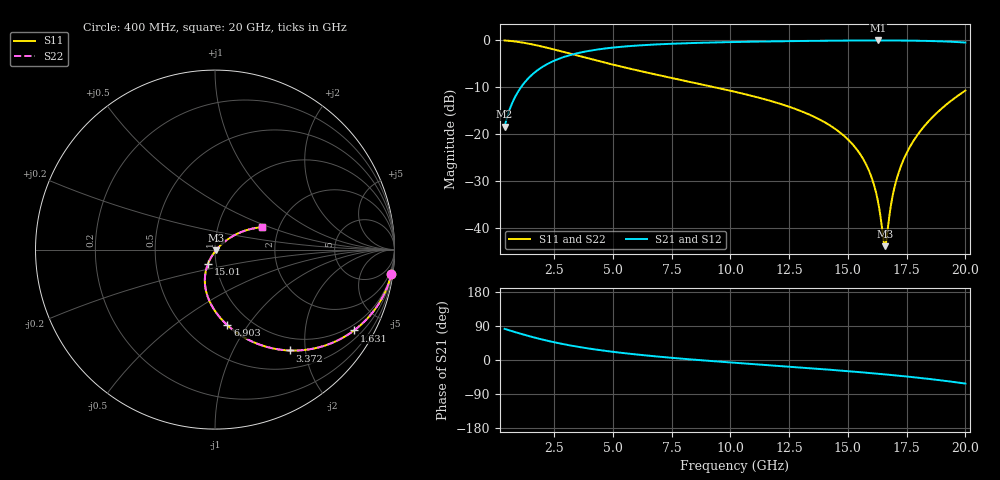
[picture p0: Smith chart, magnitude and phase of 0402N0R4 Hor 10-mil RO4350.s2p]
# GHz S MA R 50
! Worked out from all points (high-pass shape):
!   1960 points, 400 MHz to 20 GHz, reference 50 ohm
!   highest |S21| = -0.06 dB at 16.29 GHz (marker M1); lowest = -18.4 dB at 400 MHz (marker M2)
!   |S21| within 3 dB of the highest: 3.269 GHz to end of sweep
!   lowest |S11| = -43.8 dB at 16.58 GHz (marker M3), VSWR 1.01, Z = 50.5 - j0.407 ohm
!   |S11| at or under -10 dB: 9.329 GHz to end of sweep
!   |S22| runs from -43.8 to -0.1 dB; largest |S21 - S12| = 0
!   S11 on the Smith chart (normalised r, x): 400 MHz: 1, -15; 1.631 GHz: 0.78, -3.55; 3.372 GHz: 0.78, -1.71; 6.903 GHz: 0.78, -0.81; 15.01 GHz: 0.91, -0.15; 20 GHz: 1.64, +0.45
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0.4  0.9927 -7.9  0.1205 82.1  0.1205 82.1  0.9927 -7.9
0.9202654  0.9631 -17.8  0.2689 72.2  0.2689 72.2  0.9631 -17.8
1.630628  0.8962 -30.2  0.4432 59.8  0.4432 59.8  0.8962 -30.2
3.371516  0.6993 -53.5  0.7138 36.4  0.7138 36.4  0.6993 -53.5
3.671669  0.6683 -56.6  0.7428 33.3  0.7428 33.3  0.6683 -56.6
5.132414  0.5401 -69.2  0.8401 20.6  0.8401 20.6  0.5401 -69.2
6.903318  0.4272 -80.7  0.9022 9.1  0.9022 9.1  0.4272 -80.7
6.943338  0.425 -80.9  0.9032 8.9  0.9032 8.9  0.425 -80.9
10.205  0.2823 -96.9  0.9563 -7.4  0.9563 -7.4  0.2823 -96.9
13.46667  0.1573 -110.6  0.983 -22.1  0.983 -22.1  0.1573 -110.6
15.00745  0.08774 -116.2  0.9905 -29.5  0.9905 -29.5  0.08774 -116.2
15.80786  0.04596 -116.6  0.9926 -33.7  0.9926 -33.7  0.04596 -116.6
16.078  0.03085 -114.1  0.993 -35.1  0.993 -35.1  0.03085 -114.1
16.28811  0.01891 -107.4  0.993 -36.3  0.993 -36.3  0.01891 -107.4
16.50822  0.007775 -72.6  0.9929 -37.5  0.9929 -37.5  0.007775 -72.6
16.57825  0.00644 -38.8  0.9929 -38.0  0.9929 -38.0  0.00644 -38.8
16.73834  0.01207 17.9  0.9926 -38.9  0.9926 -38.9  0.01207 17.9
16.89842  0.02165 31.9  0.9923 -39.8  0.9923 -39.8  0.02165 31.9
17.09852  0.03476 37.3  0.9917 -41.0  0.9917 -41.0  0.03476 37.3
17.69883  0.07773 39.4  0.9884 -44.8  0.9884 -44.8  0.07773 39.4
18.65932  0.1569 35.1  0.9775 -51.4  0.9775 -51.4  0.1569 35.1
20  0.2911 25.4  0.9437 -62.2  0.9437 -62.2  0.2911 25.4
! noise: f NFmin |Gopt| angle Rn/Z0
0.4  0.001609  0.8892  6.174  0.003151
2.571  0.004409  0.6621  12.95  0.002466
4.752  0.006982  0.6028  16.57  0.003181
6.933  0.009541  0.5782  20.49  0.003989
9.104  0.01227  0.5711  24.48  0.004958
11.29  0.01539  0.5766  28.47  0.006227
13.47  0.01916  0.5931  32.41  0.008005
15.64  0.02395  0.6198  36.28  0.01067
17.82  0.03053  0.6571  40.18  0.01507
20  0.0403  0.7052  44.16  0.02316
